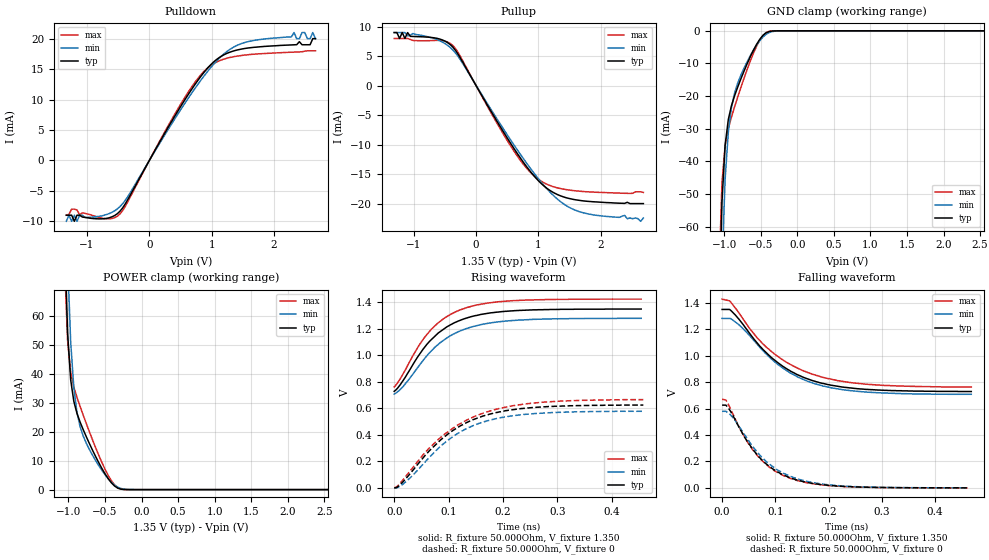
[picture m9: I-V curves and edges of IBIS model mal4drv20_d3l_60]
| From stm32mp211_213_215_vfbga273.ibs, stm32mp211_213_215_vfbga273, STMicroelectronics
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[Model] mal4drv20_d3l_60
Model_type   I/O
Polarity   Non-Inverting
Enable   Active-High
C_comp   1.902pF   1.872pF   1.915pF
C_comp_pullup   928.637fF   913.380fF   944.342fF
C_comp_pulldown   824.069fF   818.585fF   846.427fF
Vinh = 805.000mV
Vinl = 545.000mV
Vmeas = 675.000mV
Vref = 675.000mV
Rref = 50Ohms
Cref = 0pF
[Model Spec]
Vinh   805.000mV   772.000mV   855.000mV
Vinl   545.000mV   512.000mV   595.000mV
Vmeas   675.000mV   642.000mV   725.000mV
Vref   675.000mV   642.000mV   725.000mV
D_overshoot_ampl_h 0.4 NA   NA
D_overshoot_ampl_l 0.4 NA   NA
D_overshoot_area_l 110.000m NA   NA
D_overshoot_area_h 110.000m NA   NA
[Temperature Range]   25.000   125.000   -40.000
[Voltage Range]   1.350V   1.283V   1.425V
[GND Clamp Reference]   0.00V   0.00V   0.00V
[C Comp Corner]
| variable   typ   min   max
C_comp   1.902pF   1.872pF   1.915pF
C_comp_pullup   928.637fF   913.380fF   944.342fF
C_comp_pulldown   824.069fF   818.585fF   846.427fF
[Pulldown Reference]   0.00V   0.00V   0.00V
[POWER Clamp Reference]   1.350V   1.283V   1.425V
[Pullup Reference]   1.350V   1.283V   1.425V
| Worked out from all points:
|   slope of the pulldown table from 0 to 0.203 V, typ, clamps not added: 55 ohm
|   slope of the pullup table from 0 to 0.203 V, typ, clamps not added: 54.9 ohm
|   GND clamp passes 1 mA (typ) near -0.45 V on its own axis
|   POWER clamp passes 1 mA (typ) near -0.35 V on its own axis
|   rising waveform, R_fixture 50.000Ohm, V_fixture 1.350: 20-80 % time 78.1ps typ, 83.5ps min, 75.4ps max; typ from 0.728 V to 1.35 V
|   rising waveform, R_fixture 50.000Ohm, V_fixture 0: 20-80 % time 104ps typ, 102ps min, 114ps max; typ from -0.001 V to 0.624 V
|   falling waveform, R_fixture 50.000Ohm, V_fixture 1.350: 20-80 % time 102ps typ, 103ps min, 111ps max; typ from 1.35 V to 0.729 V
|   falling waveform, R_fixture 50.000Ohm, V_fixture 0: 20-80 % time 75.6ps typ, 80.4ps min, 73.6ps max; typ from 0.626 V to 0 V
[GND Clamp]
-1.332V   -728mA     -688mA     -718.9mA
-1.074V   -89.22mA   -115mA     -76.03mA
-1.031V   -52.27mA   -71.45mA   -46.39mA
-988mV    -34.98mA   -45.32mA   -35.1mA
-945mV    -27.21mA   -31.15mA   -29.98mA
-902mV    -22.97mA   -23.56mA   -26.45mA
-859.1mV  -19.9mA    -19.1mA    -23.3mA
-773.2mV  -14.75mA   -13.57mA   -17.39mA
-601.4mV  -5.967mA   -5.934mA   -6.902mA
-429.5mV  -634uA     -1.09mA    -554.5uA
-214.8mV  -1.1uA     -11.75uA   -194.3nA
2.663V    35.59nA    706.2nA    31.73nA
[Power Clamp]
-1.313V   833mA      802.3mA    823.6mA
-1.055V   90.5mA     128mA      79.41mA
-1.012V   54.31mA    79.78mA    51.52mA
-969.5mV  37.92mA    51.03mA    40.54mA
-926.6mV  30.49mA    35.21mA    35.43mA
-883.6mV  26.34mA    26.67mA    31.87mA
-840.7mV  23.31mA    21.76mA    28.71mA
-754.8mV  18.2mA     15.96mA    22.74mA
-583mV    9.188mA    8.193mA    11.73mA
-454.1mV  3.709mA    3.692mA    4.83mA
-325.2mV  504.5uA    850uA      638.6uA
2.682V    -27.23nA   -687.9nA   -20.2nA
[Pulldown]
-1.332V   -9mA       -10mA      -9mA
-1.203V   -10mA      -9mA       -8mA
-1.16V    -9mA       -10mA      -8.141mA
-1.117V   -9mA       -9mA       -8.945mA
-687.3mV  -9.52mA    -8.892mA   -9.582mA
-472.5mV  -8.359mA   -7.598mA   -8.809mA
558.4mV   9.786mA    9.215mA    10.18mA
1.031V    16.18mA    15.8mA     15.89mA
1.546V    18.41mA    19.42mA    17.32mA
2.32V     18.99mA    21mA       17.79mA
2.362V    19.01mA    20mA       17.8mA
2.663V    20mA       20mA       18mA
[Pullup]
-1.313V   9mA        9mA        8mA
-1.227V   8mA        9mA        8mA
-1.184V   9mA        9mA        8mA
-1.141V   8mA        9mA        8mA
-1.098V   9mA        8.44mA     8mA
-711.8mV  8.16mA     8.117mA    7.64mA
-368.2mV  6.483mA    5.995mA    6.753mA
576.8mV   -10.16mA   -9.571mA   -10.6mA
1.049V    -16.64mA   -16.44mA   -16.23mA
1.35V     -18.67mA   -19.64mA   -17.44mA
1.651V    -19.44mA   -21.35mA   -17.89mA
2.682V    -20mA      -22.44mA   -18.1mA
[Ramp]
R_load=50.000Ohm
dV/dt_r   374.100mV/92.000ps  345.298mV/94.000ps  399.000mV/96.000ps
dV/dt_f   374.100mV/89.500ps  345.298mV/92.500ps  399.000mV/93.000ps
[Rising waveform]
R_fixture=50.000Ohm
V_fixture=1.350
V_fixture_min=1.283
V_fixture_max=1.425
0s        728mV      707mV      761mV
17ps      813mV      767mV      864mV
41ps      974mV      896mV      1.045V
63ps      1.097V     1.01V      1.173V
75ps      1.147V     1.062V     1.224V
91ps      1.199V     1.115V     1.278V
124ps     1.269V     1.189V     1.348V
166ps     1.314V     1.238V     1.391V
229ps     1.339V     1.267V     1.415V
454ps     1.35V      1.28V      1.425V
[Rising waveform]
R_fixture=50.000Ohm
V_fixture=0
0s        -1.234mV   -1.866mV   -402.3uV
6ps       4.659mV    165.7uV    11.35mV
22ps      70.27mV    45.93mV    89.06mV
56ps      239mV      190mV      262mV
86ps      363mV      315mV      382mV
124ps     472mV      427mV      490mV
166ps     544mV      499mV      567mV
205ps     582mV      535mV      608mV
270ps     609mV      563mV      645mV
458ps     624mV      578mV      665mV
[Falling waveform]
R_fixture=50.000Ohm
V_fixture=1.350
V_fixture_min=1.283
V_fixture_max=1.425
0s        1.35V      1.282V     1.428V
14ps      1.35V      1.282V     1.415V
26ps      1.302V     1.253V     1.355V
62ps      1.115V     1.105V     1.153V
93ps      985mV      974mV      1.03V
128ps     885mV      869mV      934mV
170ps     811mV      794mV      859mV
206ps     776mV      756mV      821mV
270ps     745mV      725mV      784mV
468ps     729mV      708mV      763mV
[Falling waveform]
R_fixture=50.000Ohm
V_fixture=0
0s        626mV      579mV      670mV
7ps       626mV      579mV      665mV
19ps      557mV      538mV      570mV
47ps      353mV      372mV      350mV
66ps      249mV      269mV      244mV
96ps      141mV      157mV      135mV
127ps     77.36mV    89.11mV    73.11mV
163ps     38.28mV    45.64mV    35.97mV
227ps     11.23mV    13.96mV    9.897mV
461ps     101.7uV    176.7uV    70.77uV
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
